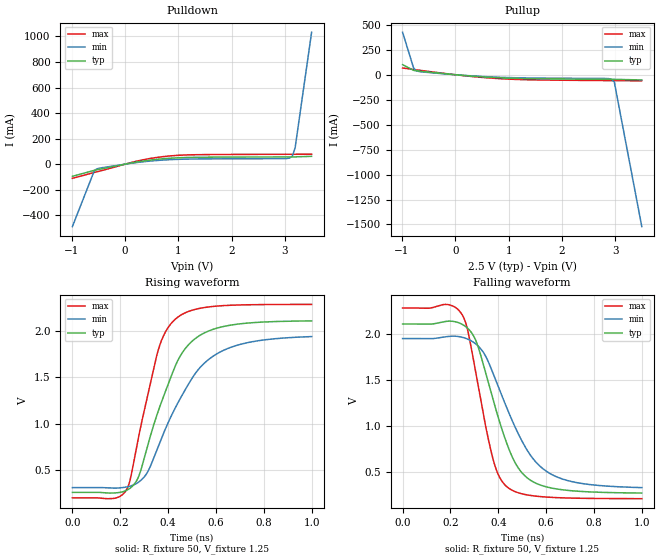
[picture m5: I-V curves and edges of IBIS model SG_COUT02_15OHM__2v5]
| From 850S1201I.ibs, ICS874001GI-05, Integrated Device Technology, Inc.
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[Model] SG_COUT02_15OHM__2v5
Model_type   Output
Polarity   Non-Inverting
|   typ   min   max
C_comp   2pF   1.5pF   2.5pF
Vmeas = 1.25V
Rref = 50
Cref = 0
Vref = 1.25V
|   typ   min   max
[Voltage range]   2.5V   2.375V   2.625V
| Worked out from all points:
|   slope of the pulldown table from 0 to 0.375 V, typ, clamps not added: 14.1 ohm
|   slope of the pullup table from 0 to 0.375 V, typ, clamps not added: 22.7 ohm
|   rising waveform, R_fixture 50, V_fixture 1.25: 20-80 % time 152ps typ, 195ps min, 110ps max; typ from 0.263 V to 2.11 V
|   falling waveform, R_fixture 50, V_fixture 1.25: 20-80 % time 133ps typ, 172ps min, 94ps max; typ from 2.11 V to 0.266 V
[Pulldown]
|Voltage   I (typ)   I (min)   I (max)
-990mV    -95.18mA   -488.6mA   -111.1mA
-577.1mV  -48.21mA   -49.44mA   -64.83mA
-525.5mV  -43.64mA   -36.24mA   -59.22mA
300.2mV   22.13mA    16.79mA    31.01mA
867.9mV   46.94mA    35.62mA    65.28mA
1.384V    53.82mA    40.8mA     74.16mA
2.984V    56.43mA    43.31mA    77.18mA
3.087V    56.54mA    47.61mA    77.29mA
3.139V    56.66mA    63.32mA    77.35mA
3.19V     56.92mA    126.8mA    77.41mA
3.5V      61.24mA    1.032A     77.82mA
[Pullup]
|Voltage   I (typ)   I (min)   I (max)
-990mV    100.9mA    425mA      67.36mA
-783.6mV  43.83mA    67.74mA    52.17mA
-732mV    39.33mA    39.44mA    48.65mA
-680.3mV  36.23mA    31.77mA    45.17mA
197mV     -9.228mA   -7.653mA   -11.74mA
867.9mV   -31.71mA   -26.24mA   -40.36mA
2.777V    -45.47mA   -37.39mA   -58.49mA
2.932V    -45.97mA   -45.22mA   -59.06mA
2.984V    -46.29mA   -73.21mA   -59.24mA
3.5V      -52.42mA   -1.521A    -61.08mA
[Ramp]
|   typ   min   max
dV/dt_r   1.479/0.238n   1.302/0.307n   1.669/0.169n
dV/dt_f   1.498/0.209n   1.32/0.274n   1.693/0.144n
R_load =   50.0000
[Rising Waveform]
R_fixture = 50
V_fixture = 1.25   |Vcc_typ
V_fixture_min = 1.1875 |Vcc_min
V_fixture_max = 1.3125 |Vcc_max
C_fixture = 0.0p
| Time   typ   min   max
0s        263mV      314.5mV    204.4mV
173.2ps   256.7mV    308.4mV    198.2mV
226.2ps   284.9mV    320.8mV    292.2mV
277.3ps   436mV      374.4mV    866.8mV
315.3ps   771.7mV    486.5mV    1.311V
359.4ps   1.14V      760.6mV    1.797V
435.4ps   1.652V     1.198V     2.136V
525.5ps   1.938V     1.58V      2.237V
620.6ps   2.039V     1.775V     2.268V
1ns       2.106V     1.937V     2.283V
[Falling Waveform]
R_fixture = 50
V_fixture = 1.25   |Vcc_typ
V_fixture_min = 1.1875 |Vcc_min
V_fixture_max = 1.3125 |Vcc_max
C_fixture = 0.0p
| Time   typ   min   max
0s        2.108V     1.95V      2.283V
188.2ps   2.139V     1.972V     2.321V
250.2ps   2.103V     1.963V     2.204V
272.3ps   2.061V     1.944V     2.039V
307.3ps   1.921V     1.888V     1.558V
377.4ps   1.293V     1.576V     642.5mV
438.4ps   787.1mV    1.177V     329.3mV
507.5ps   463.3mV    792.3mV    252.7mV
615.6ps   324.4mV    480mV      219.9mV
1ns       266.1mV    325.4mV    204.9mV
